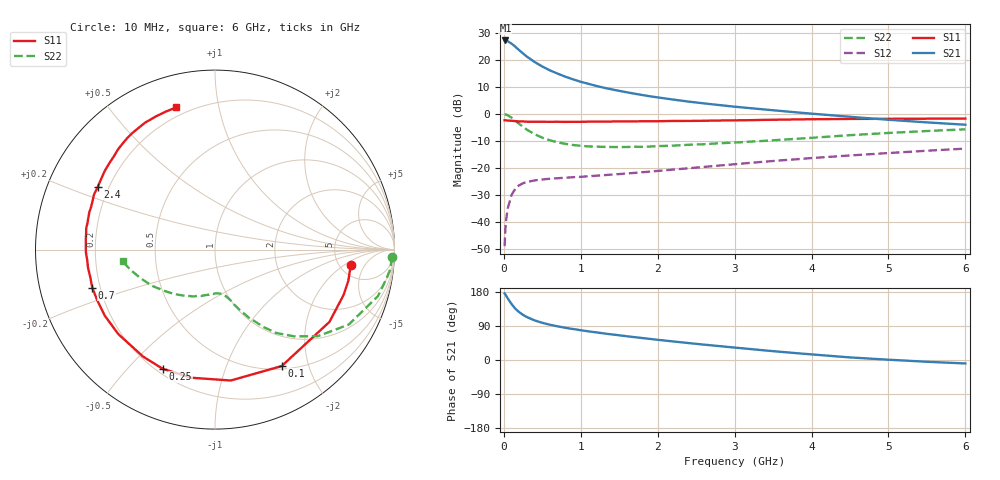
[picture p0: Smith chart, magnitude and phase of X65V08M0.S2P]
! SIEMENS Small Signal Semiconductors
! BFP193W
! Si NPN RF Bipolar Junction Transistor in SOT343
! VCE = 5 V  IC = 8 mA
! Common Emitter S-Parameters:  April 1994
# GHz  S  MA  R  50
!  f  S11  S21  S12  S22
! GHz  MAG  ANG  MAG  ANG  MAG  ANG  MAG  ANG
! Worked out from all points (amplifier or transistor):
!   40 points, 10 MHz to 6 GHz, reference 50 ohm
!   highest |S21| = 27.1 dB at 20 MHz (marker M1)
!   |S21| within 3 dB of that: start of sweep to 176.1 MHz
!   unconditionally stable (mu >= 1): 1.47 GHz to 4.233 GHz
!   at 200 MHz: K = 0.19, MSG = 25.0 dB, |S12| = -26.4 dB
!   at 1.5 GHz: K = 1.01, MAG = 14.7 dB, |S12| = -22.2 dB
!   at 6 GHz: K = 0.92, MSG = 4.4 dB, |S12| = -12.8 dB
!   lowest NFmin = 1.25 dB at 450 MHz
!   S11 on the Smith chart (normalised r, x): 10 MHz: 6.36, -2.53; 100 MHz: 0.54, -1.59; 250 MHz: 0.23, -0.63; 700 MHz: 0.17, -0.15; 2.4 GHz: 0.16, +0.25; 6 GHz: 0.15, +0.75
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0.01  0.7617 -6.3  22.71 175.6  0.0036 89.3  0.9871 -2.5
0.02  0.7628 -13.2  22.75 172.9  0.0075 82.1  0.9815 -6.7
0.03  0.7597 -19.4  22.57 169.5  0.011 80.4  0.968 -9.8
0.05  0.7542 -32.3  22.01 162.7  0.0178 74.4  0.9436 -16.0
0.1  0.7477 -60.2  19.88 147.7  0.0318 61.6  0.8538 -29.3
0.15  0.7346 -83.1  17.39 135.3  0.0416 51.7  0.7491 -40.1
0.2  0.7261 -100.5  15.02 126.1  0.048 44.9  0.6531 -47.7
0.25  0.7251 -113.6  13.09 119.0  0.0524 39.8  0.5767 -53.7
0.3  0.7183 -123.8  11.43 113.2  0.0553 36.3  0.5103 -57.8
0.4  0.7155 -138.8  9.107 104.5  0.0591 31.9  0.4214 -63.7
0.5  0.7161 -149.1  7.513 98.1  0.0615 29.9  0.3638 -67.7
0.6  0.7141 -156.6  6.361 93.0  0.0634 28.8  0.3248 -70.7
0.7  0.7159 -162.8  5.541 88.8  0.0648 28.6  0.2974 -72.8
0.9  0.7147 -172.0  4.349 81.7  0.0677 29.3  0.2664 -76.9
1.1  0.7191 -178.6  3.595 75.6  0.0705 30.7  0.2506 -80.5
1.6  0.7258 168.0  2.507 62.6  0.0795 35.8  0.2448 -89.9
2.2  0.7406 155.5  1.842 49.0  0.0935 40.6  0.2594 -102.1
2.4  0.7411 151.7  1.688 44.7  0.099 41.7  0.2687 -106.0
3.2  0.7658 137.6  1.278 29.0  0.1244 43.8  0.307 -123.1
4.5  0.8074 118.9  0.885 6.8  0.1707 41.1  0.4047 -150.1
5.5  0.8161 109.7  0.697 -4.7  0.2086 36.7  0.4829 -166.3
6  0.821 105.2  0.631 -9.1  0.2286 34.4  0.5191 -172.7
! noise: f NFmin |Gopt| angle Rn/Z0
0.45  1.25  0.23  133  0.12
0.9  1.3  0.35  156  0.11
1.8  2  0.55  -155  0.13
